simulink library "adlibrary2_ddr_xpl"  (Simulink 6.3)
undefined symbols (not defined in the file or in its folder): adlibrary2, ADM, blackbox2, blue, DDR, ddr32_config, gcbh, II, Inactive, memsize, SDRAM, Simulation, Subsystem, VER_STRING_GOES_HERE, white, xlBlockLoadCallback, XRC, XRM
libraries: xbsIndex_r4 x29, adlibrary2_ddr_xpl x1

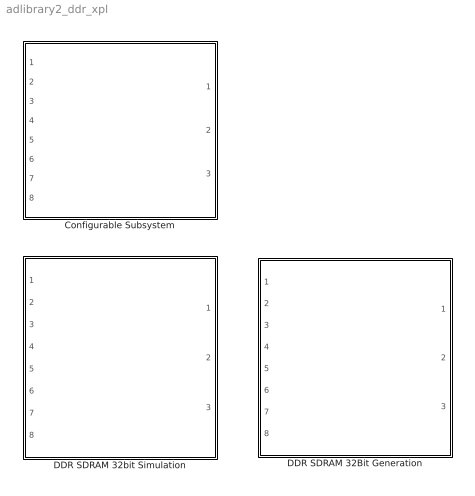
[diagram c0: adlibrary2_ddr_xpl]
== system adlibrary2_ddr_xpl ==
  Configurable Subsystem : Subsystem  Tag=configX  BlockChoice=DDR SDRAM 32bit Simulation  mask{memsize=memsize}
      mask prompts: memsize "Simulation Ram Size (Mb)"
  DDR SDRAM 32Bit Generation : Subsystem
  DDR SDRAM 32bit Simulation : Subsystem  mask{memsize=memsize}
      mask prompts: memsize "Simulation Ram Size (Mb)"

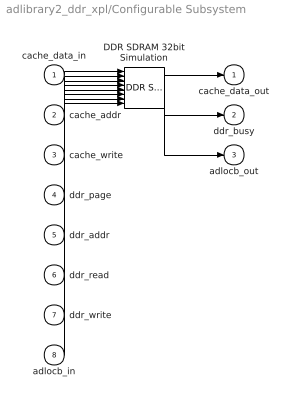
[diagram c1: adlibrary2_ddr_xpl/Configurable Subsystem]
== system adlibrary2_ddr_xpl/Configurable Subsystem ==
  cache_data_in : Inport
  cache_addr : Inport  Port=2
  cache_write : Inport  Port=3
  ddr_page : Inport  Port=4
  ddr_addr : Inport  Port=5
  ddr_read : Inport  Port=6
  ddr_write : Inport  Port=7
  adlocb_in : Inport  Port=8
  DDR SDRAM 32bit Simulation : adlibrary2_ddr_xpl/DDR SDRAM 32bit Simulation  memsize=memsize
  cache_data_out : Outport
  ddr_busy : Outport  Port=2
  adlocb_out : Outport  Port=3
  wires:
  cache_data_in/1 -> DDR SDRAM 32bit Simulation/1
  cache_addr/1 -> DDR SDRAM 32bit Simulation/2
  cache_write/1 -> DDR SDRAM 32bit Simulation/3
  ddr_page/1 -> DDR SDRAM 32bit Simulation/4
  ddr_addr/1 -> DDR SDRAM 32bit Simulation/5
  ddr_read/1 -> DDR SDRAM 32bit Simulation/6
  ddr_write/1 -> DDR SDRAM 32bit Simulation/7
  adlocb_in/1 -> DDR SDRAM 32bit Simulation/8
  DDR SDRAM 32bit Simulation/1 -> cache_data_out/1
  DDR SDRAM 32bit Simulation/2 -> ddr_busy/1
  DDR SDRAM 32bit Simulation/3 -> adlocb_out/1

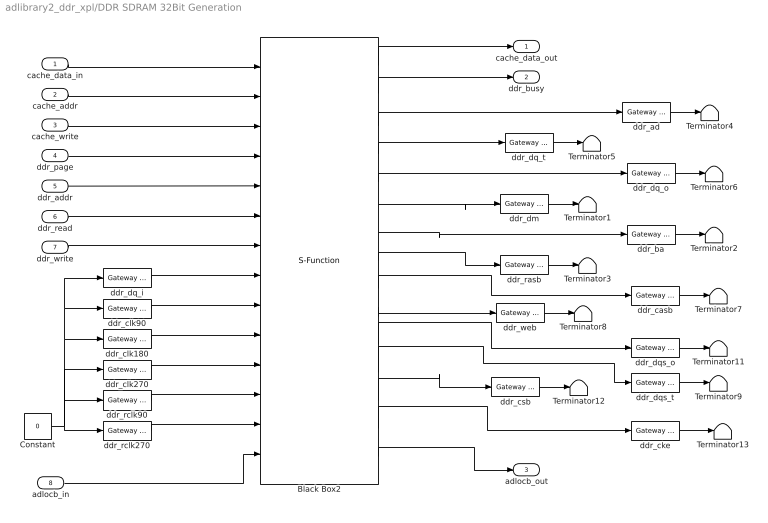
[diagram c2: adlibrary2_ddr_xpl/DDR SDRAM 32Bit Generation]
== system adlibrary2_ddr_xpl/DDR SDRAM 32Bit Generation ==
  cache_data_in : Inport
  cache_addr : Inport  Port=2
  cache_write : Inport  Port=3
  ddr_page : Inport  Port=4
  ddr_addr : Inport  Port=5
  ddr_read : Inport  Port=6
  ddr_write : Inport  Port=7
  adlocb_in : Inport  Port=8
  Black Box2 : S-Function  LoadFcn=xlBlockLoadCallback(gcbh);  FunctionName=sysgen  Parameters=ptable_  mask(Xilinx Black Box Block){infoedit=Incorporates black box HDL and simulation model into a System Generator design.<P><P>You must supply a Black Box with certain information about the HDL component you would like to bring into System Generator. This information is provided through a Matlab function.<P><P>When "Simulation mode" is set to "Inactive", you will typically want to provide a separate simulation model by using a Simulation 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, init_code=ddr32_config, sim_method=Inactive, sim_method_sgadvanced=, engine_block=, xl_use_area=off, xl_use_area_sgadvanced=, xl_area=[0,0,0,0,0,0,0], block_version=VER_STRING_GOES_HERE, has_advanced_control=0, sggui_pos=20,20,356,367, block_type=blackbox2, sg_icon_stat=135,512,14,15,white,blue,0,4aa598fc, sg_mask_display=fprintf('','COMMENT: begin icon graphics '); patch([0 130 130 0 ],[0 0 170 170 ],[0.77 0.82 0.91]); patch([31 9 39 9 31 65 74 83 120 91 63 43 74 43 63 91 120 83 74 65 31 ],[34 56 86 116 138 138 129 138 138 109 137 117 86 55 35 63 34 34 43 34 34 ],[0.98 0.96 0.92]); plot([0 0 130 130 0 ],[0 170 170 0 0 ]); fprintf('','COMMENT: end icon graphics');  fprintf('','COMMENT: begin icon text '); color('bl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, sg_list_contents=, adlocb_devid=1, ddr_size=64}
      mask prompts: infoedit ""; init_code "Block configuration m-function"; sim_method "Simulation mode"; engine_block "HDL co-simulator to use  (specify helper block by name)"; xl_use_area "Define FPGA area for resource estimation"; xl_area "FPGA area [slices, FFs, BRAMs, LUTs, IOBs, emb. mults, TBUFs]"; block_version ""; has_advanced_control ""; sggui_pos ""; block_type ""; sg_icon_stat ""; sg_mask_display ""; sg_list_contents ""; adlocb_devid "ADLOCB DEV ID"; ddr_size "DDR BANK SIZE"
      mask help: Incorporates black box HDL and simulation model into a System Generator design. You must supply a Black Box with certain information about the HDL component you would like to bring into System Generator. This information is provided through a Matlab function. When "Simulation mode" is set to "Inactive", you will typically want to provide a separate simulation model by using a Simulation Multiplexer. When "Simulation mode" is set to "External co-simulator", you must include a ModelSim block in the design.
      mask init:
      | xlMungeMaskParams;
      | 
      | mdlPath = xlGetMdlDir(bdroot);
      | 
      | refBlk = get_param(gcb,'referenceBlock');
      | if (isempty(refBlk) | strncmp(refBlk,'xbsIndex',8))
      | srcPath = mdlPath;
      | else
      | srcPath = xlPathToReference;
      | if (isempty(srcPath))
      | srcPath = mdlPath;
      | end
      | end
      | 
      | if (sim_method==3)
      | validEngineBlock = 0;
      | try
      | engineBlock = xlBlockNameRelPath(get_param(gcb,'Parent'),engine_block);
      | catch
      | engineBlock = '//';
      | end
      | try 
      | engineWorkDir = get_param(engineBlock,'dir');
      | validEngineBlock = 1;
      | engine_handle = get_param(engineBlock,'Handle');
      | catch
      | end
      | end
      | 
      | % build black box config function
      | block_config = ['sysgen:black_box_config:' init_code];
      | 
      | serialized_declarations = '{''engine_handle''=>''Double'',''sim_method''=>''Int'',''validEngineBlock''=>''Int'',''engineWorkDir''=>''String'',''engine_block''=>''String'',''init_code''=>''String'',''mdlPath''=>''String'',''srcPath''=>''String'',''block_config''=>''String'',}';
      | ptable_ = xlblockprep(get_param(gcb, 'MaskWSVariables'));
  Constant : Constant  Value=0
  Terminator{1..9,11..13} (12 alike) : Terminator
  ddr_ad : xbsIndex_r4/Gateway Out  hdl_port=on  timing_constraint=None  locs_specified=off  LOCs={}  block_type=gatewayout
  ddr_ba : xbsIndex_r4/Gateway Out  hdl_port=on  timing_constraint=None  locs_specified=off  LOCs={}  block_type=gatewayout
  ddr_casb : xbsIndex_r4/Gateway Out  hdl_port=on  timing_constraint=None  locs_specified=off  LOCs={}  block_type=gatewayout
  ddr_cke : xbsIndex_r4/Gateway Out  hdl_port=on  timing_constraint=None  locs_specified=off  LOCs={}  block_type=gatewayout
  ddr_clk180 : xbsIndex_r4/Gateway In  arith_type=Boolean  n_bits=64  bin_pt=0  period=1  dbl_ovrd=off  timing_constraint=None  locs_specified=off  LOCs={}  block_type=gatewayin
  ddr_clk270 : xbsIndex_r4/Gateway In  arith_type=Boolean  n_bits=64  bin_pt=0  period=1  dbl_ovrd=off  timing_constraint=None  locs_specified=off  LOCs={}  block_type=gatewayin
  ddr_clk90 : xbsIndex_r4/Gateway In  arith_type=Boolean  n_bits=64  bin_pt=0  period=1  dbl_ovrd=off  timing_constraint=None  locs_specified=off  LOCs={}  block_type=gatewayin
  ddr_csb : xbsIndex_r4/Gateway Out  hdl_port=on  timing_constraint=None  locs_specified=off  LOCs={}  block_type=gatewayout
  ddr_dm : xbsIndex_r4/Gateway Out  hdl_port=on  timing_constraint=None  locs_specified=off  LOCs={}  block_type=gatewayout
  ddr_dq_i : xbsIndex_r4/Gateway In  arith_type=Unsigned  n_bits=32  bin_pt=0  period=1  dbl_ovrd=off  timing_constraint=None  locs_specified=off  LOCs={}  block_type=gatewayin
  ddr_dq_o : xbsIndex_r4/Gateway Out  hdl_port=on  timing_constraint=None  locs_specified=off  LOCs={}  block_type=gatewayout
  ddr_dq_t : xbsIndex_r4/Gateway Out  hdl_port=on  timing_constraint=None  locs_specified=off  LOCs={}  block_type=gatewayout
  ddr_dqs_o : xbsIndex_r4/Gateway Out  hdl_port=on  timing_constraint=None  locs_specified=off  LOCs={}  block_type=gatewayout
  ddr_dqs_t : xbsIndex_r4/Gateway Out  hdl_port=on  timing_constraint=None  locs_specified=off  LOCs={}  block_type=gatewayout
  ddr_rasb : xbsIndex_r4/Gateway Out  hdl_port=on  timing_constraint=None  locs_specified=off  LOCs={}  block_type=gatewayout
  ddr_rclk270 : xbsIndex_r4/Gateway In  arith_type=Boolean  n_bits=64  bin_pt=0  period=1  dbl_ovrd=off  timing_constraint=None  locs_specified=off  LOCs={}  block_type=gatewayin
  ddr_rclk90 : xbsIndex_r4/Gateway In  arith_type=Boolean  n_bits=64  bin_pt=0  period=1  dbl_ovrd=off  timing_constraint=None  locs_specified=off  LOCs={}  block_type=gatewayin
  ddr_web : xbsIndex_r4/Gateway Out  hdl_port=on  timing_constraint=None  locs_specified=off  LOCs={}  block_type=gatewayout
  cache_data_out : Outport
  ddr_busy : Outport  Port=2
  adlocb_out : Outport  Port=3
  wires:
  ddr_cke/1 -> Terminator13/1
  ddr_csb/1 -> Terminator12/1
  ddr_dqs_o/1 -> Terminator11/1
  ddr_web/1 -> Terminator8/1
  ddr_casb/1 -> Terminator7/1
  ddr_rasb/1 -> Terminator3/1
  ddr_ba/1 -> Terminator2/1
  ddr_dm/1 -> Terminator1/1
  ddr_dq_o/1 -> Terminator6/1
  ddr_dq_t/1 -> Terminator5/1
  ddr_ad/1 -> Terminator4/1
  Black Box2/2 -> ddr_busy/1
  Black Box2/1 -> cache_data_out/1
  ddr_write/1 -> Black Box2/7
  ddr_read/1 -> Black Box2/6
  ddr_addr/1 -> Black Box2/5
  ddr_page/1 -> Black Box2/4
  cache_write/1 -> Black Box2/3
  cache_addr/1 -> Black Box2/2
  cache_data_in/1 -> Black Box2/1
  ddr_dq_i/1 -> Black Box2/8
  Constant/1 -> ddr_dq_i/1, ddr_clk90/1, ddr_clk180/1, ddr_rclk270/1, ddr_clk270/1, ddr_rclk90/1
  ddr_clk90/1 -> Black Box2/9
  ddr_clk180/1 -> Black Box2/10
  ddr_clk270/1 -> Black Box2/11
  ddr_rclk90/1 -> Black Box2/12
  ddr_rclk270/1 -> Black Box2/13
  ddr_dqs_t/1 -> Terminator9/1
  Black Box2/3 -> ddr_ad/1
  Black Box2/4 -> ddr_dq_t/1
  Black Box2/5 -> ddr_dq_o/1
  Black Box2/6 -> ddr_dm/1
  Black Box2/7 -> ddr_ba/1
  Black Box2/8 -> ddr_rasb/1
  Black Box2/9 -> ddr_casb/1
  Black Box2/10 -> ddr_web/1
  Black Box2/11 -> ddr_dqs_o/1
  Black Box2/12 -> ddr_dqs_t/1
  Black Box2/13 -> ddr_csb/1
  Black Box2/14 -> ddr_cke/1
  adlocb_in/1 -> Black Box2/14
  Black Box2/15 -> adlocb_out/1

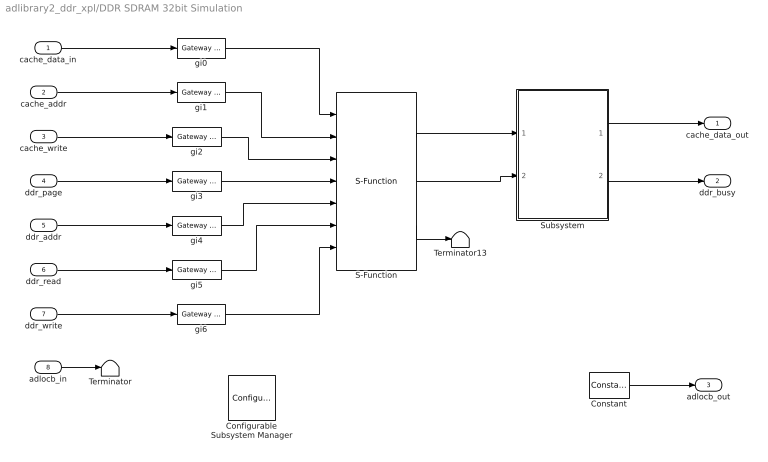
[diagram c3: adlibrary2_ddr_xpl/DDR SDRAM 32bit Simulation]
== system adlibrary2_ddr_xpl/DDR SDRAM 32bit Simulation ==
  cache_data_in : Inport
  cache_addr : Inport  Port=2
  cache_write : Inport  Port=3
  ddr_page : Inport  Port=4
  ddr_addr : Inport  Port=5
  ddr_read : Inport  Port=6
  ddr_write : Inport  Port=7
  adlocb_in : Inport  Port=8
  Configurable Subsystem Manager : xbsIndex_r4/Configurable Subsystem Manager  Tag=xcfgMgr  block_type=configsubsys
  Constant : xbsIndex_r4/Constant  arith_type=Unsigned  const=0  n_bits=66  bin_pt=0  explicit_period=on  period=1  equ=P=C  opselect=C  inp2=PCIN>>17  opr=+  inp1=P  carry=CIN  dbl_ovrd=off  block_type=constant
  S-Function : S-Function  FunctionName=ddr32  Parameters=memsize,0
  Subsystem : Subsystem  AncestorBlock=adlibrary2/ADM-XRC-II/XRM DDR SDRAM /DDR SDRAM 64bit Simulation/Subsystem
  Terminator : Terminator
  Terminator13 : Terminator
  gi{0..6} (7 alike) : xbsIndex_r4/Gateway Out  hdl_port=off  timing_constraint=None  locs_specified=off  LOCs={}  block_type=gatewayout
  cache_data_out : Outport
  ddr_busy : Outport  Port=2
  adlocb_out : Outport  Port=3
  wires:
  cache_data_in/1 -> gi0/1
  cache_addr/1 -> gi1/1
  cache_write/1 -> gi2/1
  ddr_page/1 -> gi3/1
  ddr_addr/1 -> gi4/1
  ddr_read/1 -> gi5/1
  ddr_write/1 -> gi6/1
  gi0/1 -> S-Function/1
  gi1/1 -> S-Function/2
  gi2/1 -> S-Function/3
  gi3/1 -> S-Function/4
  gi4/1 -> S-Function/5
  gi5/1 -> S-Function/6
  gi6/1 -> S-Function/7
  S-Function/2 -> Subsystem/2(In2)
  S-Function/1 -> Subsystem/1(In1)
  Subsystem/1(Out1) -> cache_data_out/1
  Subsystem/2(Out2) -> ddr_busy/1
  S-Function/3 -> Terminator13/1
  Constant/1 -> adlocb_out/1
  adlocb_in/1 -> Terminator/1

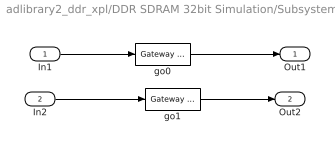
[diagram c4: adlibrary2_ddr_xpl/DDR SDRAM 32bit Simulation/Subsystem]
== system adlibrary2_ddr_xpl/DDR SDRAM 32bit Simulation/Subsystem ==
  In1 : Inport
  In2 : Inport  Port=2
  go0 : xbsIndex_r4/Gateway In  arith_type=Unsigned  n_bits=32  bin_pt=0  period=1  dbl_ovrd=off  timing_constraint=None  locs_specified=off  LOCs={}  block_type=gatewayin
  go1 : xbsIndex_r4/Gateway In  arith_type=Boolean  n_bits=32  bin_pt=0  period=1  dbl_ovrd=off  timing_constraint=None  locs_specified=off  LOCs={}  block_type=gatewayin
  Out1 : Outport
  Out2 : Outport  Port=2
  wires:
  go1/1 -> Out2/1
  go0/1 -> Out1/1
  In2/1 -> go1/1
  In1/1 -> go0/1
